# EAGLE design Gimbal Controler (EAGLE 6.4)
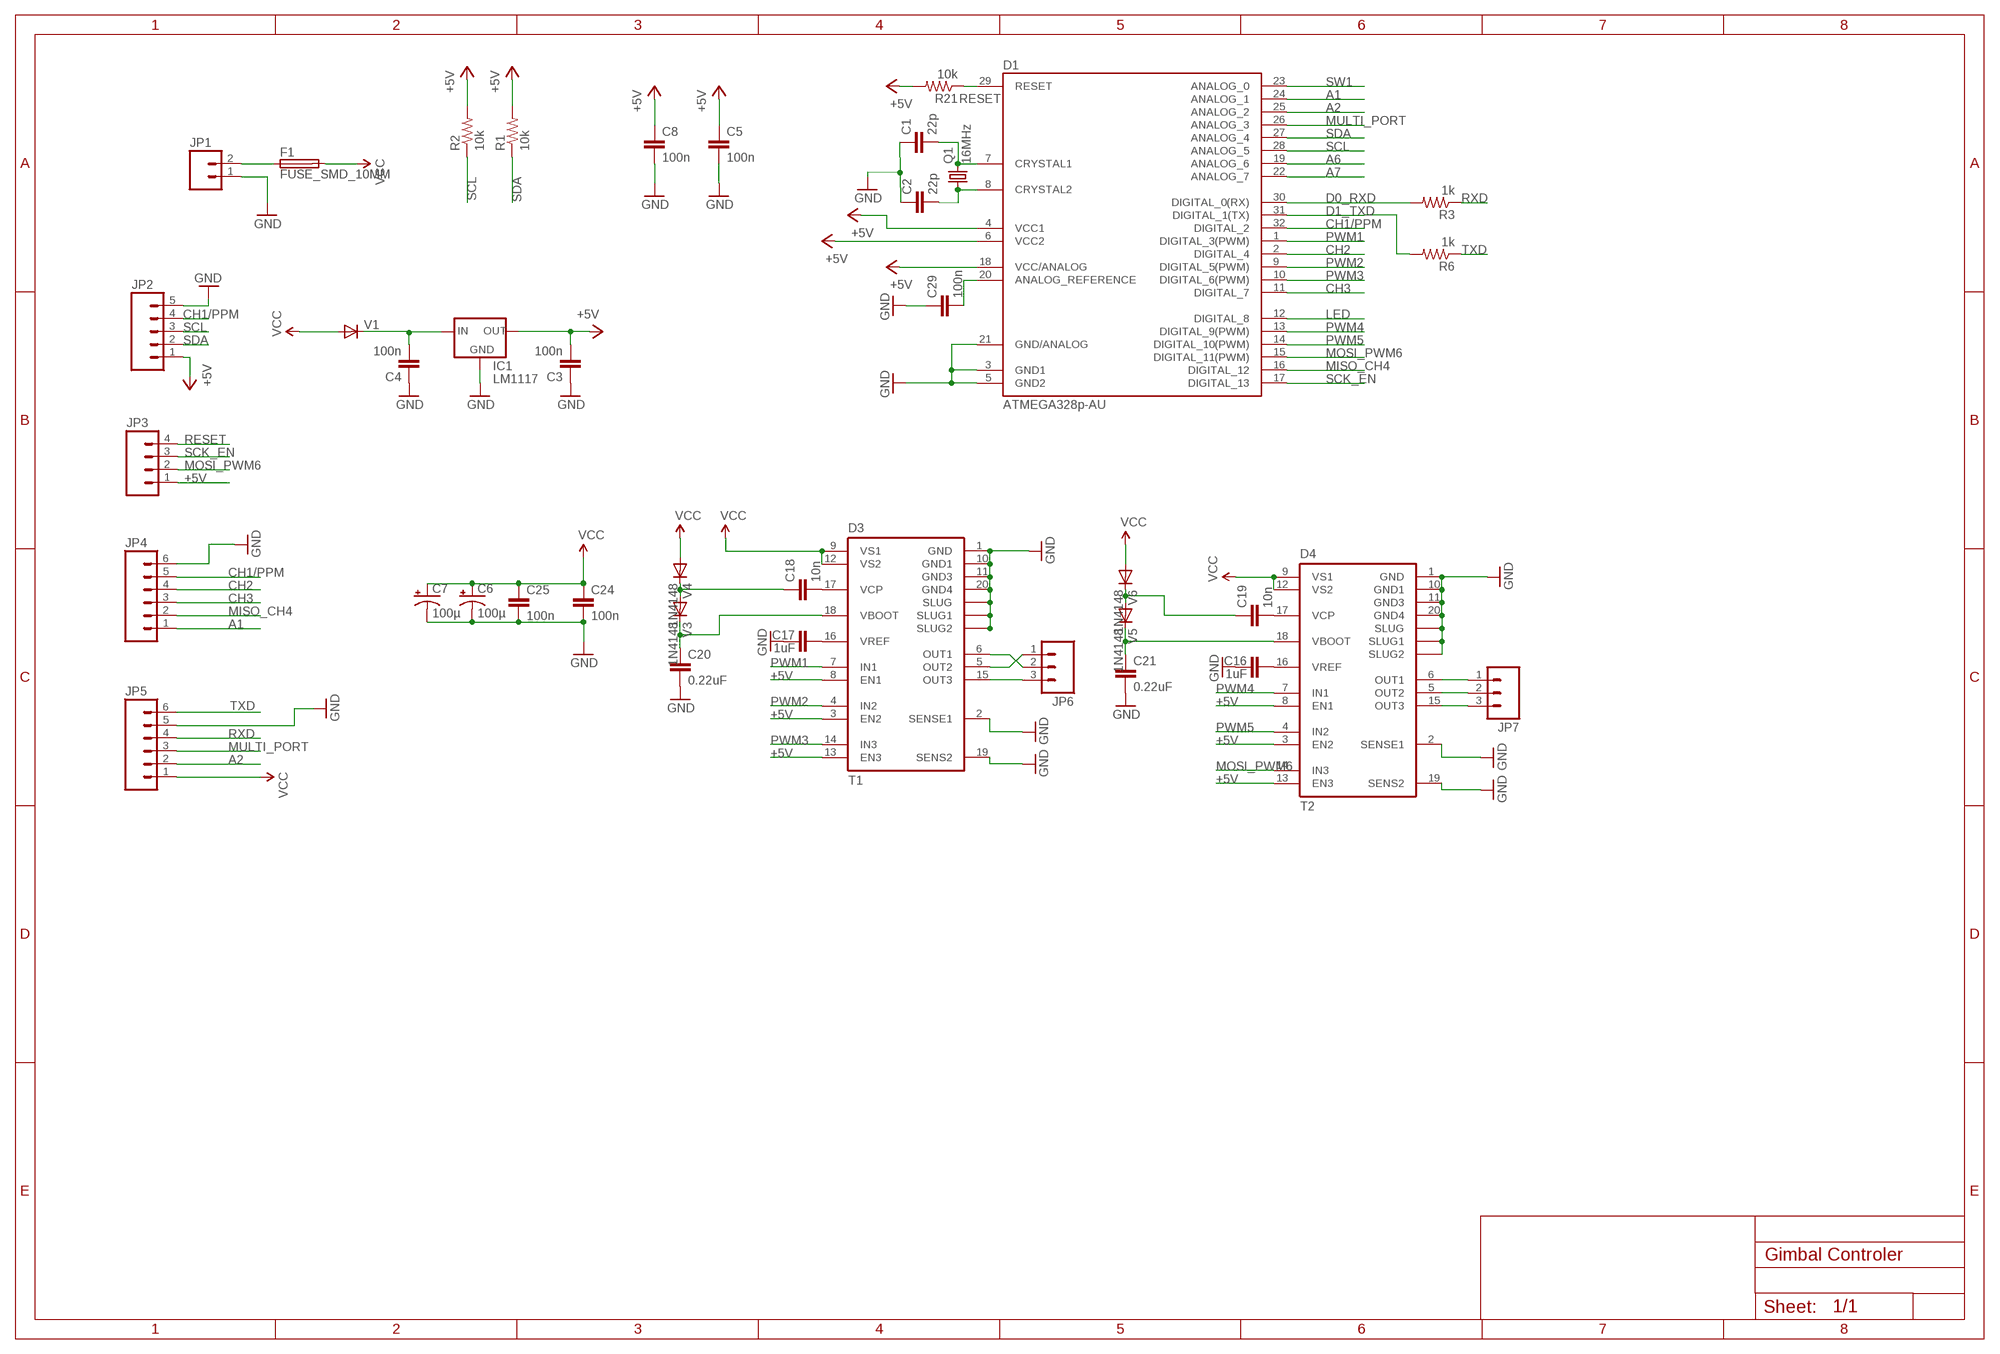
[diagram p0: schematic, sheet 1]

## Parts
C1  22p  CAP0805  [0805]
C2  22p  CAP0805  [0805]
C3  100n  CAP0805  [0805]
C4  100n  CAP0805  [0805]
C5  100n  CAP0805  [0805]
C6  100µ  CAP_POLD  [PANASONIC_D]
C7  100µ  CAP_POLD  [PANASONIC_D]
C8  100n  CAP0805  [0805]
C16  1uF  CAP0805  [0805]
C17  1uF  CAP0805  [0805]
C18  10n  CAP0805  [0805]
C19  10n  CAP0805  [0805]
C20  0.22uF  CAP0805  [0805]
C21  0.22uF  CAP0805  [0805]
C24  100n  CAP0805  [0805]
C25  100n  CAP0805  [0805]
C29  100n  CAP0805  [0805]
D1  ATMEGA328p-AU  ATMEGA168-AU  [TQFP32-08]
D3  T1  L6234  [SO20POWER2]
D4  T2  L6234  [SO20POWER2]
F1  FUSE_SMD_10MM  [SMD_FUSE_10MM]
IC1  LM1117  [SOT223]
JP1  M02PTH  [1X02]
JP2  M05PTH  [1X05]
JP3  M04PTH  [1X04]
JP4  M06SIP  [1X06]
JP5  M06SIP  [1X06]
JP6  M03PTH  [1X03]
JP7  M03PTH  [1X03]
Q1  16MHz  CRYSTALHC49S  [HC49/S]
R1  10k  RESISTOR0805-RES  [0805]
R2  10k  RESISTOR0805-RES  [0805]
R3  1k  RESISTOR0805-RES  [0805]
R6  1k  RESISTOR0805-RES  [0805]
R21  10k  RESISTOR0805-RES  [0805]
V1  DIODE-DO214AC  [DO214AC]
V3  1N4148  DIODE-MINIMELF  [MINIMELF]
V4  1N4148  DIODE-MINIMELF  [MINIMELF]
V5  1N4148  DIODE-MINIMELF  [MINIMELF]
V6  1N4148  DIODE-MINIMELF  [MINIMELF]

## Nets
+5V: C3.2 C5.1 C8.1 D1.4(VCC1) D1.6(VCC2) D1.18(VCC/ANALOG) D3.3(EN2) D3.8(EN1) D3.13(EN3) D4.3(EN2) D4.8(EN1) D4.13(EN3) IC1.2(OUT) JP2.1 JP3.1 R1.2 R2.2 R21.2
A1: D1.24(ANALOG_1) JP4.1
A2: D1.25(ANALOG_2) JP5.2
A6: D1.19(ANALOG_6)
A7: D1.22(ANALOG_7)
CH1/PPM: D1.32(DIGITAL_2) JP2.4 JP4.5
CH2: D1.2(DIGITAL_4) JP4.4
CH3: D1.11(DIGITAL_7) JP4.3
D0_RXD: D1.30(DIGITAL_0(RX)) R3.2
D1_TXD: D1.31(DIGITAL_1(TX)) R6.2
GND: C1.1 C2.1 C3.1 C4.1 C5.2 C6.- C7.- C8.2 C16.1 C17.1 C20.2 C21.2 C24.2 C25.2 C29.1 D1.3(GND1) D1.5(GND2) D1.21(GND/ANALOG) D3.1(GND) D3.2(SENSE1) D3.10(GND1) D3.11(GND3) D3.19(SENS2) D3.20(GND4) D3.SLUG1(SLUG2) D3.SLUG2(SLUG) D3.SLUG(SLUG1) D4.1(GND) D4.2(SENSE1) D4.10(GND1) D4.11(GND3) D4.19(SENS2) D4.20(GND4) D4.SLUG1(SLUG2) D4.SLUG2(SLUG) D4.SLUG(SLUG1) IC1.1(GND) JP1.1 JP2.5 JP4.6 JP5.5
LED: D1.12(DIGITAL_8)
MISO_CH4: D1.16(DIGITAL_12) JP4.2
MOSI_PWM6: D1.15(DIGITAL_11(PWM)) D4.14(IN3) JP3.2
MULTI_PORT: D1.26(ANALOG_3) JP5.3
N$3: F1.P$1 JP1.2
N$7: C16.2 D4.16(VREF)
N$8: C17.2 D3.16(VREF)
N$17: C18.2 D3.17(VCP)
N$18: C19.2 D4.17(VCP)
N$19: C19.1 V5.A V6.C
N$20: C21.1 D4.18(VBOOT) V5.C
N$21: D3.15(OUT3) JP6.3
N$23: D4.6(OUT1) JP7.1
N$24: D4.5(OUT2) JP7.2
N$25: D4.15(OUT3) JP7.3
N$27: D3.5(OUT2) JP6.1
N$28: D3.6(OUT1) JP6.2
N$38: C2.2 D1.8(CRYSTAL2) Q1.1
N$39: C1.2 D1.7(CRYSTAL1) Q1.2
N$40: C29.2 D1.20(ANALOG_REFERENCE)
PWM1: D1.1(DIGITAL_3(PWM)) D3.7(IN1)
PWM2: D1.9(DIGITAL_5(PWM)) D3.4(IN2)
PWM3: D1.10(DIGITAL_6(PWM)) D3.14(IN3)
PWM4: D1.13(DIGITAL_9(PWM)) D4.7(IN1)
PWM5: D1.14(DIGITAL_10(PWM)) D4.4(IN2)
RESET: D1.29(RESET) JP3.4 R21.1
RXD: JP5.4 R3.1
SCK_EN: D1.17(DIGITAL_13) JP3.3
SCL: D1.28(ANALOG_5) JP2.3 R2.1
SDA: D1.27(ANALOG_4) JP2.2 R1.1
SW1: D1.23(ANALOG_0)
TXD: JP5.6 R6.1
VBOOT1: C20.1 D3.18(VBOOT) V3.C
VCC: C6.+ C7.+ C24.1 C25.1 D3.9(VS1) D3.12(VS2) D4.9(VS1) D4.12(VS2) F1.P$2 JP5.1 V1.A V4.A V6.A
VCC_VI: C4.2 IC1.3(IN) V1.C
VCP1: C18.1 V3.A V4.C

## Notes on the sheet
- FTDI

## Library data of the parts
C1-C5 C8 C16-C21 C24 C25 C29 = SparkFun:CAP: Capacitor
C6 C7 = SparkFun:CAP_POL: Capacitor Polarized
D1 = Arduino-AVR:ATMEGA168
D3 D4 = L6234:L6234
F1 = f-lf-omniblok-s:FUSE_SMD_10MM
IC1 = v-reg-2:LM1117
JP1 = SparkFun:M02: Header 2
JP2 = SparkFun:M05: Header 5 Standard 5-pin 0.1" header. Use with straight break away headers (SKU : PRT-00116), right angle break away headers (PRT-00553), swiss pins (PRT-00743), machine pins (PRT-00117), and female headers (PRT-00115). Molex polarized connector foot print use with SKU : PRT-08230 with associated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
JP3 = SparkFun:M04: Header 4 Standard 4-pin 0.1" header. Use with straight break away headers (SKU : PRT-00116), right angle break away headers (PRT-00553), swiss pins (PRT-00743), machine pins (PRT-00117), and female headers (PRT-00115). Molex polarized connector foot print use with SKU : PRT-08231 with associated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
JP4 JP5 = SparkFun:M06: Header 6 Standard 6-pin 0.1" header. Use with straight break away headers (SKU : PRT-00116), right angle break away headers (PRT-00553), swiss pins (PRT-00743), machine pins (PRT-00117), and female headers (PRT-00115). Molex polarized connector foot print use with SKU : PRT-08094 with associated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
JP6 JP7 = SparkFun:M03: Header 3 Standard 3-pin 0.1" header. Use with straight break away headers (SKU : PRT-00116), right angle break away headers (PRT-00553), swiss pins (PRT-00743), machine pins (PRT-00117), and female headers (PRT-00115). Molex polarized connector foot print use with SKU : PRT-08232 with associated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
Q1 = crystal:CRYSTAL: CRYSTAL; OC_FARNELL: 1667008; OC_NEWARK: unknown
R1-R3 R6 R21 = SparkFun:RESISTOR: Resistor
V1 V3-V6 = diode:DIODE-: DIODE

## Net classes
0 default: width 0.406 mm, clearance 0.152 mm

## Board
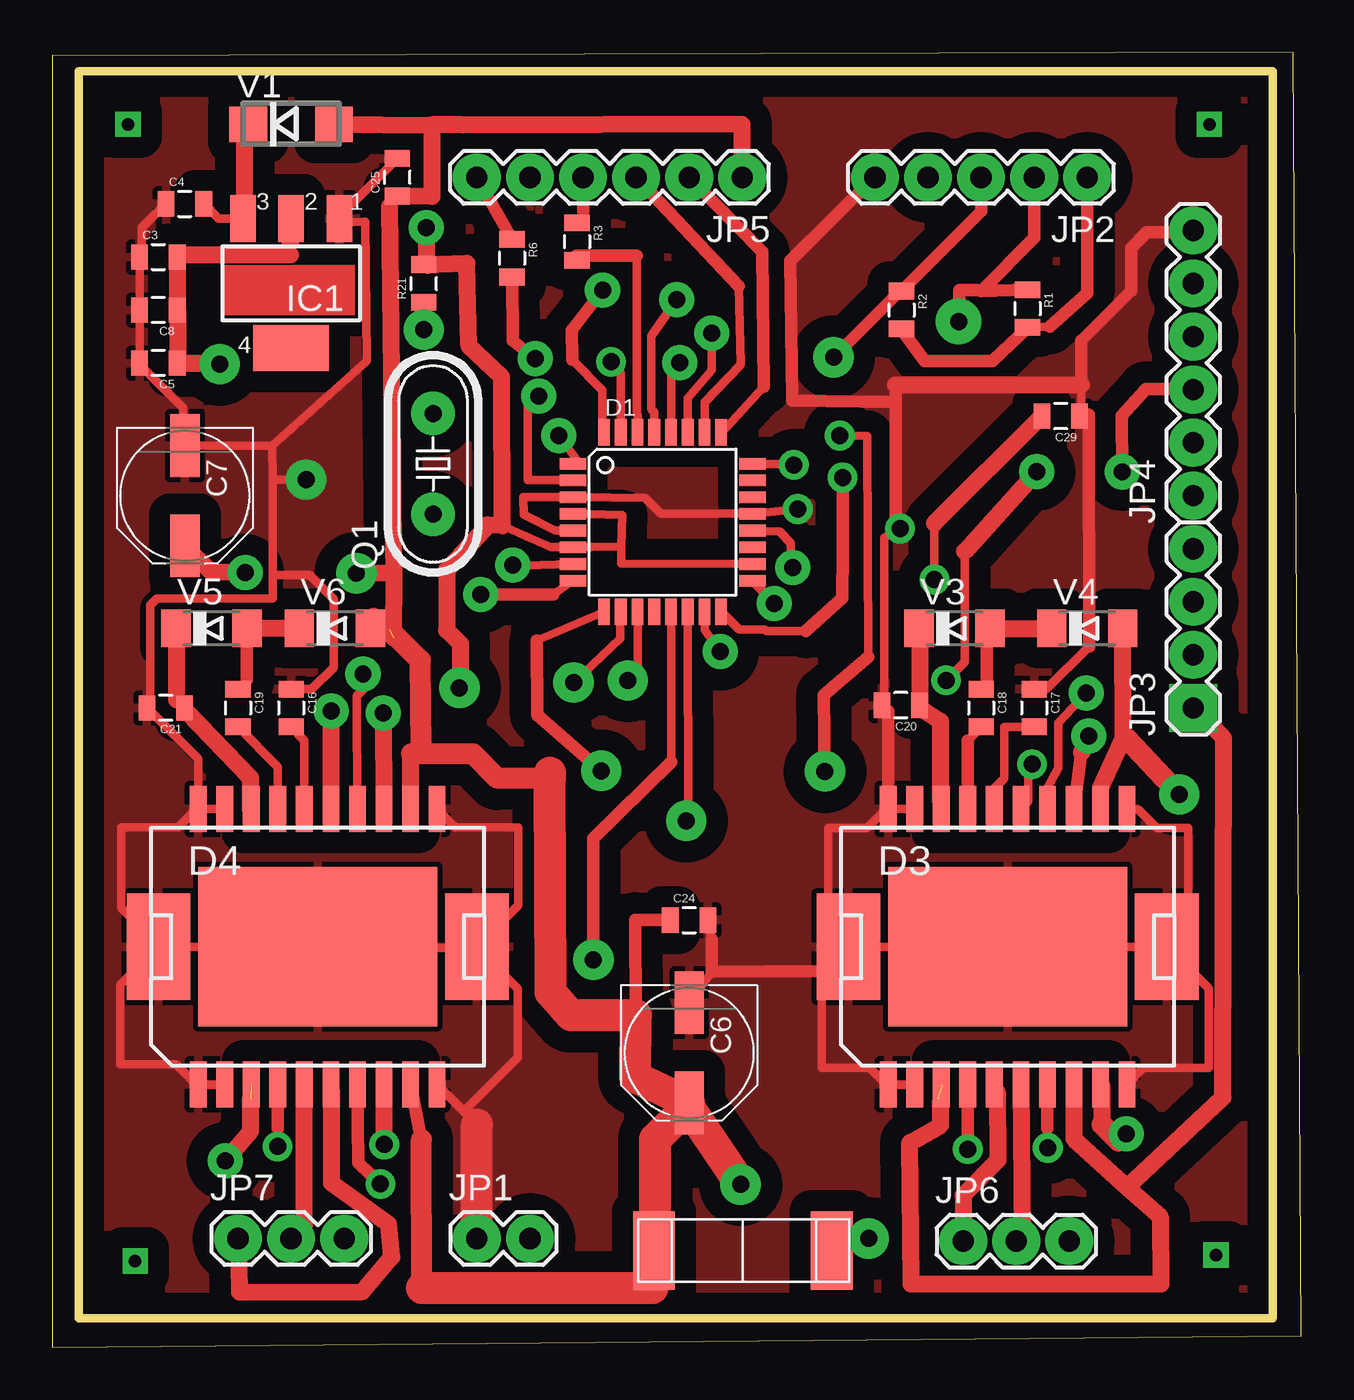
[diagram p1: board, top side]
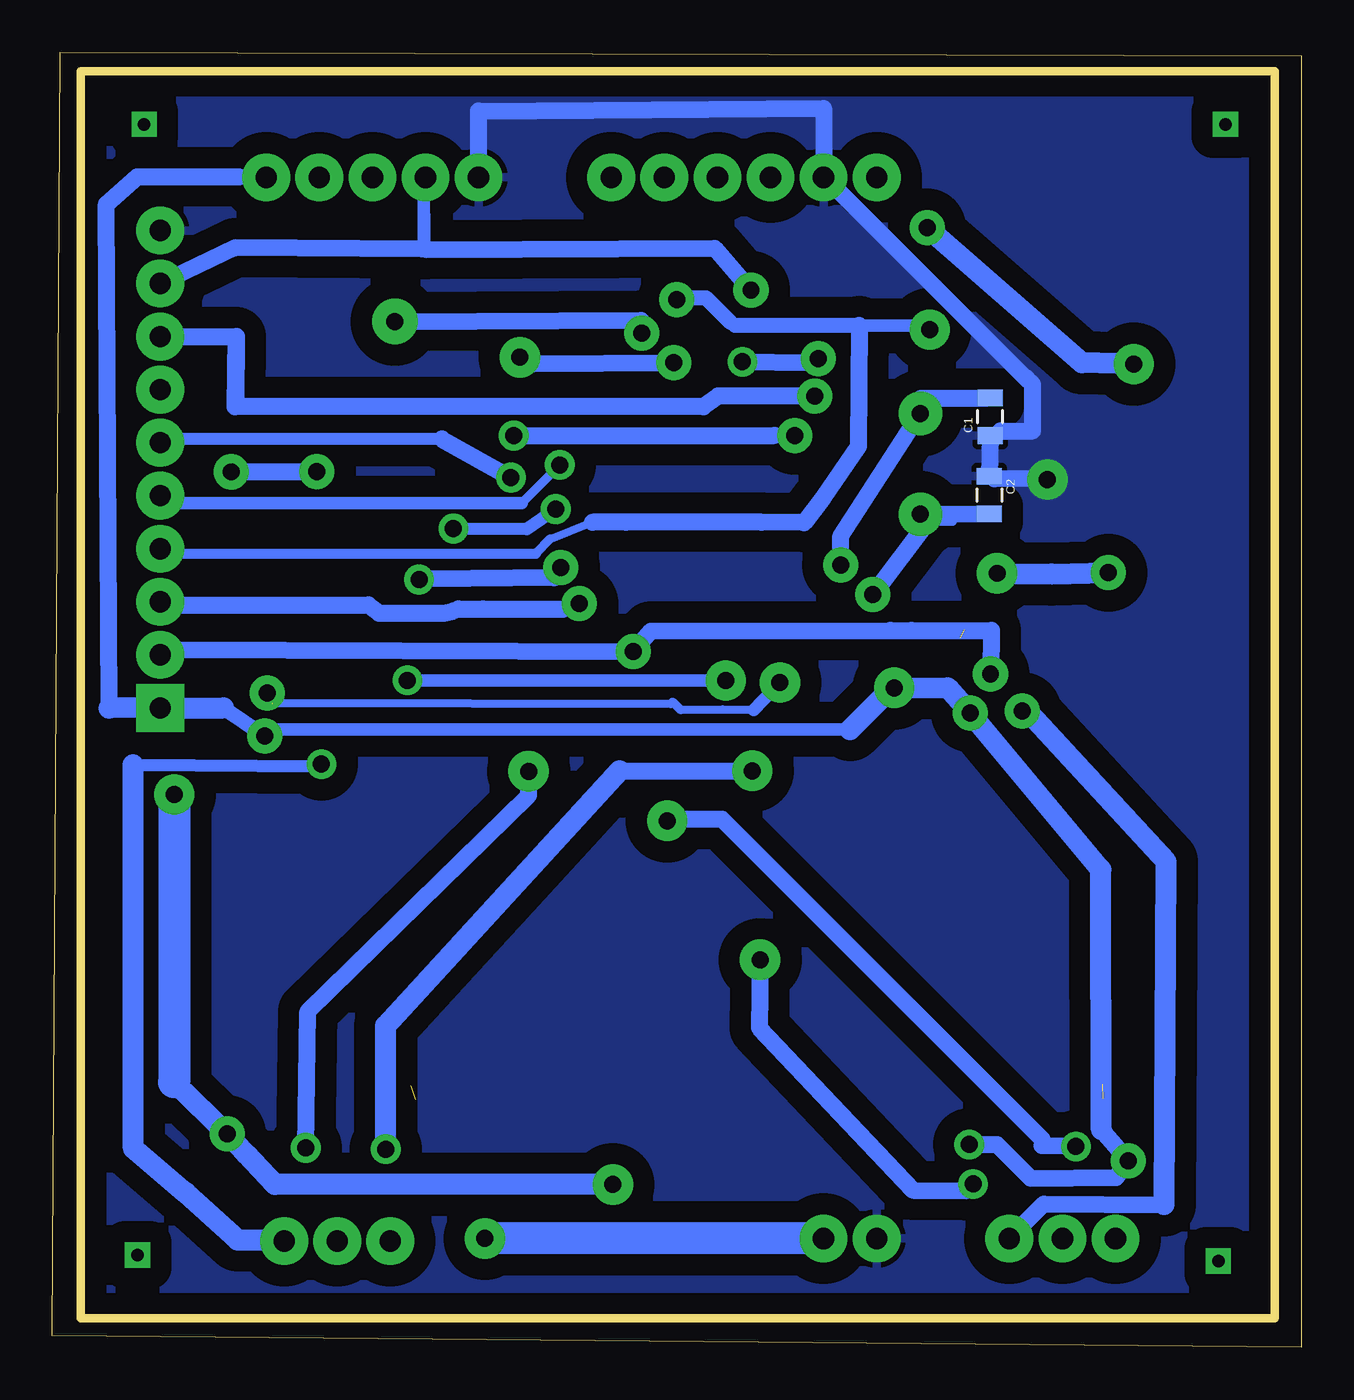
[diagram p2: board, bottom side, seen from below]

Size 59.77 x 62 mm. Coordinates in mm from the lower left corner, seen from the top.
Outline: 0,0 59.77,0.54 59.39,62 0,61.84 0,0
Outline: 58.42,61.09 58.42,1.4 1.27,1.4 1.27,61.09 58.42,61.09
Copper layers (1*16): Top 0.035mm / dielectric 1.5mm / Bottom 0.035mm
Design rules "default": minimum track width 10mil, minimum drill 32mil, track to track 12mil, track to pad 12mil, pad to pad 12mil, via to via 12mil, smd to smd 8mil, copper to edge 40mil, drill to drill 40mil, minimum pad ring 25mil, minimum via ring 12mil, stop-mask expansion 4mil, vias tented up to drill 0mil, thermal gap 10mil

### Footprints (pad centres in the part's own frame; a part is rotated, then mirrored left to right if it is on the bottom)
0805 = smd 0.8 x 1.2: 1 -0.9,0; 2 0.9,0
PANASONIC_D = smd 3 x 1.4: + 2.4,0; - -2.4,0
TQFP32-08 = smd 1.27 x 0.559: 1 -4.293,2.8; 2 -4.293,2; 3 -4.293,1.2; 4 -4.293,0.4; 5 -4.293,-0.4; 6 -4.293,-1.2; 7 -4.293,-2; 8 -4.293,-2.8; 17 4.293,-2.8; 18 4.293,-2; 19 4.293,-1.2; 20 4.293,-0.4; 21 4.293,0.4; 22 4.293,1.2; 23 4.293,2; 24 4.293,2.8 | smd 0.559 x 1.27: 9 -2.8,-4.293; 10 -2,-4.293; 11 -1.2,-4.293; 12 -0.4,-4.293; 13 0.4,-4.293; 14 1.2,-4.293; 15 2,-4.293; 16 2.8,-4.293; 25 2.8,4.293; 26 2,4.293; 27 1.2,4.293; 28 0.4,4.293; 29 -0.4,4.293; 30 -1.2,4.293; 31 -2,4.293; 32 -2.8,4.293
SO20POWER2 = smd 0.8 x 2.2: 1 -5.715,-6.6; 2 -4.445,-6.6; 3 -3.175,-6.6; 4 -1.905,-6.6; 5 -0.635,-6.6; 6 0.635,-6.6; 7 1.905,-6.6; 8 3.175,-6.6; 9 4.445,-6.6; 10 5.715,-6.6; 11 5.715,6.6; 12 4.445,6.6; 13 3.175,6.6; 14 1.905,6.6; 15 0.635,6.6; 16 -0.635,6.6; 17 -1.905,6.6; 18 -3.175,6.6; 19 -4.445,6.6; 20 -5.715,6.6 | smd 3.048 x 5.08: SLUG -7.62,0; SLUG2 7.62,0 | smd 11.43 x 7.62: SLUG1 0,0
SMD_FUSE_10MM = smd 2 x 3.75: P$1 4.25,0; P$2 -4.25,0
SOT223 = smd 1.219 x 2.235: 1 -2.311,-3.099; 2 0,-3.099; 3 2.311,-3.099 | smd 3.6 x 2.2: 4 0,3.099
1X02 = drill 1.016 pad 1.88: 1 0,0; 2 2.54,0
1X05 = drill 1.016 pad 1.88: 1 0,0; 2 2.54,0; 3 5.08,0; 4 7.62,0; 5 10.16,0
1X04 = drill 1.016 pad 1.88 square: 1 0,0 | drill 1.016 pad 1.88: 2 2.54,0; 3 5.08,0; 4 7.62,0
1X06 = drill 1.016 pad 1.88: 1 0,0; 2 2.54,0; 3 5.08,0; 4 7.62,0; 5 10.16,0; 6 12.7,0
1X03 = drill 1.016 pad 1.88: 1 0,0; 2 2.54,0; 3 5.08,0
HC49/S = drill 0.813: 1 -2.413,0; 2 2.413,0
DO214AC = smd 1.8 x 1.7: A 2.05,0; C -2.05,0
MINIMELF = smd 1.4 x 1.8: A 1.7,0; C -1.7,0

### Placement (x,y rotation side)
C1  14.89,44.55 90 bottom
C2  14.92,40.8 270 bottom
C3  5.08,52.2 0 top
C4  6.35,54.74 0 top
C5  5.08,47.12 180 top
C6  30.48,14.1 270 top
C7  6.35,40.77 270 top
C8  5.08,49.66 180 top
C16  11.43,30.61 270 top
C17  46.99,30.61 270 top
C18  44.45,30.61 270 top
C19  8.89,30.61 270 top
C20  40.61,30.73 180 top
C21  5.43,30.61 180 top
C24  30.48,20.45 0 top
C25  16.51,56.01 90 top
C29  48.26,44.58 180 top
D1  29.21,39.5 0 top
D3  45.72,19.18 0 top
D4  12.7,19.18 0 top
F1  33.05,4.64 0 top
IC1  11.43,50.93 180 top
JP1  20.32,5.21 0 top
JP2  49.53,56.01 180 top
JP3  54.61,30.61 90 top
JP4  54.61,40.77 90 top
JP5  33.02,56.01 180 top
JP6  43.59,5.08 0 top
JP7  8.89,5.21 0 top
Q1  18.22,42.29 90 top
R1  46.67,49.72 270 top
R2  40.64,49.66 270 top
R3  25.11,52.93 270 top
R6  22,52.13 270 top
R21  17.78,50.93 90 top
V1  11.43,58.55 0 top
V3  43.18,34.42 0 top
V4  49.53,34.42 0 top
V5  7.62,34.42 0 top
V6  13.53,34.42 0 top

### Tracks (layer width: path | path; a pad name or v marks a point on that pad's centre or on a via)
+5V  (via drill 0.81, 0.81 pad 1.68, 0.81 pad 1.93)  (2 unrouted)
  Top 0.406: 40.64,48.74 R2.2 | 47.73,48.86 R1.2 | 48.97,26.23 D3.13 | 42.6,12.52 D3.3 | 5.99,47.12 C5.1 | 5.99,49.66 C8.1 5.99,49.84 | 5.99,52.2 C3.2 6.17,52.3 | 11.41,52.9 IC1.2 11.49,53.81 | 11.41,52.3 11.38,52.84 | 21.54,39.33 22.71,38.8 23.85,38.3 D1.6 25.09,38.3 25.78,38.3 25.79,38.32 | R21.2 17.95,51.8 | 27.23,38.33 27.27,39.84 D1.4 | 25.79,38.32 27.23,38.33 | 27.23,38.33 27.23,38.34 25.79,38.32 | 27.23,38.33 27.23,37.52 D1.18 | 8.02,47.12 v8.02,47.07 | 41.04,9.8 41.14,9.84 | 42.51,11.75 42.39,11.88 | 19.53,31.61 v19.48,31.57
  Top 0.61: 40.64,48.74 41.75,47.22 44.99,47.22 R1.2 | 47.73,48.86 49.53,50.47 JP2.1 | 49.25,28.46 48.97,26.23
  Top 0.813: v49.6,29.25 49.25,28.46 | 41.04,9.8 41.1,3.02 53.05,3.02 53.02,6.27 51.45,7.65 | 51.45,7.65 48.9,9.98 D3.8 | JP3.1 56.06,29.16 56.03,11.94 51.45,7.65 | v15.89,9.71 15.87,10.49 D4.8 | v15.84,30.36 D4.13 | 5.99,49.66 5.99,47.12 8.02,47.12 | 5.99,49.84 5.99,52.2 | 11.38,52.84 11.41,52.9 | 6.17,52.3 11.41,52.3 | R21.2 19.84,51.89 19.93,47.94 21.51,46.46 21.54,39.33 20.84,39.36 18.88,37.21 18.88,34.33 19.53,33.69 19.53,31.61 | 17.95,51.8 v17.9,53.61 | 41.14,9.84 42.51,10.64 42.51,11.75 | v8.29,8.92 9.49,10.34 9.49,11.91
  Bottom 0.406: 50.83,56.04 JP2.1 | 54.62,30.63 JP3.1 | v15.89,9.71 15.87,9.19 | 49.4,29.57 49.84,29.13 v49.6,29.25 | 19.66,31.5 v19.48,31.57 | 8.87,8.13 v8.29,8.92
  Bottom 0.61: 21.59,29.57 49.4,29.57
  Bottom 0.711: 51.59,30.61 v49.6,29.25
  Bottom 0.813: 50.83,56.04 55.71,56.04 57.18,54.72 57.05,30.59 | 8.85,8.14 v8.29,8.92 9.56,10.41 | v15.89,9.71 14.57,9.71 12.95,8.1 8.87,8.13
  Bottom 1.016: JP3.1 51.59,30.61 | 54.62,30.63 57.05,30.59 | 9.56,10.41 9.6,22.87 v15.84,30.36 16.93,31.58 v19.48,31.57 | 19.66,31.5 21.59,29.57 | v8.02,47.07 10.5,47.13 v17.9,53.61
A1  (via drill 0.81)
  Top 0.406: v35.48,42.24 35.48,42.29 D1.24
  Bottom 0.406: 37.31,40.41 v35.48,42.24 | JP4.1 54.25,40.41
  Bottom 0.61: 54.25,40.41 37.31,40.41
A2
  Top 0.406: 34.06,45.98 32.03,43.79 D1.25
  Top 0.61: 34.06,45.98 33.97,52.46 JP5.2
CH1/PPM  (via drill 0.81 pad 1.68)
  Top 0.406: 24.89,47.28 26.31,45.82 26.31,43.87 26.39,43.79 D1.32
  Top 0.61: 24.89,47.28 24.86,48.7 v26.33,50.62
  Bottom 0.406: 41.88,52.55 JP2.4 42.09,55.91 42.08,52.58
  Bottom 0.813: v26.33,50.62 28.07,52.61 41.88,52.55 | JP4.5 51.02,52.64 42.08,52.58
CH2  (via drill 0.81 pad 1.68)
  Top 0.406: v23.28,45.54 22.76,45.14 22.76,41.5 D1.2
  Bottom 0.813: JP4.4 50.96,48.39 | 50.96,48.39 51,45.19 | v23.28,45.54 27.9,45.54 28.61,45.02 51.02,45.02 50.96,48.39
CH3  (via drill 0.81, 0.81 pad 1.68, 0.81 pad 1.93)
  Top 0.406: v27.54,31.92 28.02,32.28 D1.11 | v42.77,31.93 43.66,32.82 43.66,38.09 | 54.58,45.88 JP4.3
  Top 0.61: v51.21,41.91 51.18,44.61 52.32,45.88 54.58,45.88
  Top 0.813: v47.1,41.92 43.66,38.09
  Bottom 0.406: 28.12,31.93 v27.54,31.92
  Bottom 0.61: v42.77,31.93 28.12,31.93
  Bottom 0.813: v47.1,41.92 48.27,41.91 v51.21,41.91
D0_RXD
  Top 0.406: 25.07,52.25 25.05,52.04 R3.2 | 27.97,52.25 27.97,44.68 28.02,44.63 D1.30
  Top 0.61: 27.97,52.25 25.07,52.25
D1_TXD  (via drill 0.81, 0.81 pad 1.68)
  Top 0.406: v26.75,47.18 27.2,46.66 D1.31
  Top 0.61: v23.11,47.32 22.03,48.2 R6.2
  Bottom 0.813: v23.11,47.32 23.66,47.15 v26.75,47.18
GND  (via drill 0.81, 0.81 pad 1.93)
  Top 0.406: 49.62,33.54 47.57,31.52 46.99,31.52 C17.1 | 49.59,44.64 C29.1 49.25,44.76 49.25,46.08 | D3.SLUG2 55.35,17.17 55.35,13.39 52.22,13.39 51.44,12.6 D3.10 | D3.11 51.44,25.76 51.97,25.76 52.86,24.87 54.36,24.87 54.36,20.27 53.44,19.36 D3.SLUG2 | D3.SLUG2 D3.SLUG1 D3.SLUG | D1.5 24.08,39.09 22.57,39.87 22.54,40.7 24.05,40.69 D1.3 25.09,40.69 28.39,40.66 28.87,40.18 29.12,39.9 D1.21 33.68,39.9 v35.68,40.13 | 40.01,30.45 39.73,30.73 C20.2 39.83,30.91 39.83,38.76 v40.58,39.19 40.36,39.37 | D3.19 40.18,25.78 D3.20 39.83,25.68 39.01,24.87 37.14,24.87 37.14,18.64 D3.SLUG | 31.56,19.53 31.37,20.45 C24.2 | C6.- 31.56,17.98 | D3.2 D3.1 39.83,12.68 39.12,13.39 36.83,13.39 36.83,17.91 D3.SLUG | 36.65,18.01 D3.SLUG | 20.32,10.67 19.7,11.29 | 19.7,11.29 D4.10 | D4.SLUG2 22.3,21.16 22.3,24.89 19.28,24.89 18.41,25.76 D4.11 | 19.7,11.29 22.28,13.87 22.28,17.14 20.42,19 D4.SLUG2 | D4.20 6.98,28.17 4.55,30.61 C21.2 4.65,30.79 4.7,30.84 4.7,35.54 5,35.84 10.54,35.84 10.54,37.02 | D4.19 7.16,25.78 D4.20 | D4.2 D4.1 6.81,12.68 5.94,13.54 3.25,13.54 3.25,17.35 D4.SLUG | D4.20 6.81,25.68 6.02,24.89 3.3,24.89 3.3,21.03 4.98,19.36 D4.SLUG | D4.SLUG D4.SLUG1 12.88,19.13 20.12,19.13 D4.SLUG2 | C4.1 5.44,54.74 4.29,53.59 4.29,52.38 C3.1 4.19,52.2 4.19,49.84 C8.2 4.19,49.66 4.19,47.12 C5.2 4.29,46.94 6.27,44.96 6.27,43.36 C7.- 6.35,43.16 10.53,43.17 | C25.2 16.51,56.9 13.74,54.13 IC1.1 13.84,53.85 14.99,53.88 15.05,47.21 10.53,43.17 | 10.54,41.54 10.54,37.02 | 10.53,43.17 10.54,41.54 | 11.43,31.52 C16.1 12.42,31.51 13.46,32.54 13.46,35.81 12.32,36.96 10.6,36.96 10.54,37.02 | v12.15,41.54 10.54,41.54
  Top 0.406: 40.31,45.26 40.36,46.08 | 54.52,53.37 JP4.6
  Top 0.61: 49.59,44.64 49.62,33.54 | 49.25,46.08 49.25,48.2 51.63,50.58 51.63,52.61 52.39,53.37 54.52,53.37 | D3.20 40.01,30.45 | 31.56,19.53 31.56,17.98 36.65,18.01 | 40.36,39.37 40.36,46.08 | 40.31,45.26 35.41,45.32 35.31,52.01 JP2.5
  Top 0.813: 40.36,46.08 49.25,46.08
  Top 1.524: JP1.1 20.32,10.67
  Bottom 0.406: v12.15,41.54 11.88,41.57 | 14.68,41.58 C2.1 | 13.16,46.41 13.18,46.41 | 22.68,55.91 JP5.5 | 14.4,43.87 C1.1
  Bottom 0.61: v35.68,40.13 37.06,39.16 v40.58,39.19
  Bottom 0.813: JP5.5 22.86,59.31 39.37,59.18 JP2.5 | C1.1 C2.1 | 11.88,41.57 14.68,41.58 | 13.18,46.41 22.68,55.91 | 13.16,46.41 12.85,46.1 12.85,43.87 14.4,43.87
  pour Bottom (isolate 1.016): 1.43,61.02 58.23,61.12 58.42,60.93 58.45,1.37 1.33,1.27 1.24,1.37 1.24,60.83
  pour Top (isolate 1.016): 58.36,61.15 58.42,58.71 58.32,4.03 58.36,1.62 1.4,1.59 1.21,1.4 1.3,61.09
  pour Bottom (isolate 1.016): 58.39,61.02 58.36,57.88 58.36,57.4 58.42,41.91 58.45,1.49 58.36,1.46 1.4,1.52 0.86,60.99 2,60.99
MISO_CH4  (via drill 0.81)
  Top 0.406: 36.07,34.29 34.16,34.29 34.09,34.37 32.87,34.37 32.03,35.2 D1.16
  Top 0.61: 36.07,34.29 37.81,35.87 37.82,38.12 v37.82,41.63
  Bottom 0.406: JP4.2 54.05,43.51
  Bottom 0.61: 54.05,43.51 41.13,43.48
  Bottom 0.813: 41.13,43.48 v37.82,41.63
MOSI_PWM6  (via drill 0.81 pad 1.68)
  Top 0.406: v31.97,33.31 31.22,34.34 D1.15 | D4.14 14.57,31.18 14.87,31.49 v14.87,32.23
  Bottom 0.406: 18.64,34.32 19.67,34.32 | JP3.2 54.1,33.4
  Bottom 0.813: 18.64,34.32 31.12,34.28 v31.97,33.31 54.1,33.4 | 19.67,34.32 14.83,34.32 v14.87,32.23
MULTI_PORT
  Top 0.406: 32.84,50.79 32.94,47.05 31.22,45.24 D1.26
  Top 0.61: JP5.3 32.84,50.79
N$1  (via drill 0.6)
  other vias: 3.97,4.13
N$2  (via drill 0.6)
  other vias: 55.69,4.41
N$3  (via drill 0.81 pad 1.93)
  Top 0.406: v39.07,5.21 F1.P$1
  Bottom 1.524: JP1.2 v39.07,5.21
N$4  (via drill 0.6)
  other vias: 55.37,58.55
N$5  (via drill 0.6)
  other vias: 3.62,58.55
N$7
  Top 0.406: D4.16 12.06,29.06 11.43,29.69 C16.2
N$8
  Top 0.406: D3.16 45.09,26.75 45.57,27.23 45.57,29.69 46.99,29.69 C17.2
N$17
  Top 0.406: 43.82,29.06 44.45,29.69 C18.2
  Top 0.61: D3.17 43.82,29.06
N$18
  Top 0.406: D4.17 10.79,27.79 8.89,29.69 C19.2
N$19
  Top 0.406: 9.32,31.94 C19.1
  Top 0.61: V5.A 9.32,31.94
  Top 0.813: V6.C V5.A
N$20
  Top 0.406: 5.94,30.99 C21.1 6.43,30.43 | 5.94,34.42 V5.C | 9.49,25.72 D4.18
  Top 0.813: 5.94,34.42 5.94,30.99 | 9.49,25.72 9.49,27.27 6.43,30.43
N$21  (via drill 0.81)
  Top 0.406: v46.89,27.91 46.71,27.74 46.71,26.14 D3.15
  Bottom 0.406: 46.99,27.81 v46.89,27.91 | 53.41,7.4 53.37,7.4 | 48.74,5.14 JP6.3
  Bottom 0.61: 55.91,27.88 46.99,27.81
  Bottom 1.016: 55.91,27.88 55.89,9.51 53.41,7.4 | 53.37,7.4 50.9,5.14 48.74,5.14
N$23
  Top 0.406: 13.37,12.25 D4.6
  Top 0.813: 13.37,12.25 13.37,7.85 16.1,5.89 16.26,4.33 14.85,2.67 8.95,2.63 JP7.1
N$24
  Top 0.813: D4.5 12.06,5.84 JP7.2
N$25  (via drill 0.81 pad 1.68)
  Top 0.406: 13.33,26.17 D4.15 | 13.33,27.9 13.33,27.84
  Top 0.813: 13.33,27.84 13.33,26.17 | 13.33,27.9 13.33,29.24 v13.34,30.45
  Bottom 0.406: 13.02,30.35 v13.34,30.45
  Bottom 0.813: 6.56,6.83 12.32,6.86 JP7.3
  Bottom 1.016: 13.02,30.35 6.46,23.25 6.56,6.83
N$27
  Top 0.406: 45.22,12.25 D3.5
  Top 0.813: 45.22,12.25 45.25,8.96 43.59,7.27 JP6.1
N$28
  Top 0.406: 46.42,5.3 JP6.2
  Top 0.813: D3.6 46.42,5.3
N$38  (via drill 0.81 pad 1.68)
  Top 0.406: 23.97,36.04 D1.8
  Top 0.61: v20.51,36.04 23.97,36.04
  Bottom 0.406: 15.22,39.91 15.08,39.92 C2.2 | 17.88,39.52 16.69,39.52 Q1.1
  Bottom 0.813: Q1.1 15.22,39.91 | 17.88,39.52 v20.51,36.04
N$39  (via drill 0.81 pad 1.68)
  Top 0.406: v22.03,37.45 22.57,37.43 D1.7
  Bottom 0.406: Q1.2 18.19,45.43 | 15.08,45.43 C1.2
  Bottom 0.813: 18.19,45.43 15.08,45.43 | v22.03,37.45 22.06,38.78 Q1.2
N$40  (via drill 0.81, 0.81 pad 1.68)
  Top 0.406: v42.22,36.75 42.22,39.45 | v35.43,37.34 35.34,38.02 35.34,38.49 34.81,39.06 D1.20 | 47.35,44.58 C29.2
  Top 0.813: 42.22,39.45 47.35,44.58
  Bottom 0.406: 41.74,36.79 v42.22,36.75
  Bottom 0.813: 41.74,36.79 35.76,36.85 v35.43,37.34
PWM1  (via drill 0.81, 0.81 pad 1.68, 0.81 pad 1.93)
  Top 0.406: v24.24,43.64 25.09,42.49 24.92,42.32 D1.1 | v37.69,43.65 39.01,43.63 39.04,33.04 | 47.62,10.49 v47.64,9.55
  Top 0.61: 39.04,33.04 36.91,31.23 v36.98,27.57 | D3.7 47.62,10.49
  Bottom 0.406: 25.22,43.65 v24.24,43.64
  Bottom 0.813: v37.69,43.65 25.22,43.65 | v36.98,27.57 36.98,26.42 47.54,16.08 v47.64,9.55
PWM2  (via drill 0.81, 0.81 pad 1.93)
  Top 0.406: 23.19,33.85 26.39,35.2 D1.9
  Top 0.61: 23.19,33.85 23.22,30.27 v26.28,27.6 | D3.4 v43.82,9.49
  Bottom 0.813: 32.63,27.6 v26.28,27.6
  Bottom 1.016: 32.63,27.6 43.82,15.39 v43.82,9.49
PWM3  (via drill 0.81 pad 1.68, 0.81 pad 1.93)  (1 unrouted)
  Top 0.406: v24.95,31.83 27.17,33.92 D1.10 | v49.49,31.32 48.14,29.88 48.14,27.74 47.62,26.75 D3.14
  Bottom 0.406: v49.49,31.32 49.24,30.83 | 26.2,30.51 27.69,30.54 29.69,30.51 30.07,30.89 30.1,30.89 30.19,30.81 49.27,30.84
  Bottom 0.61: 26.2,30.51 v24.95,31.83
PWM4  (via drill 0.81, 0.81 pad 1.93)
  Top 0.406: 29.62,28.02 D1.13
  Top 0.61: 29.62,28.02 25.9,24.36 v25.9,18.55 | v15.7,7.82 14.64,8.82 D4.7
  Bottom 0.813: v25.9,18.55 25.93,15.29 18.57,7.52 16.03,7.49 v15.7,7.82
PWM5  (via drill 0.81, 0.81 pad 1.93)
  Top 0.406: v30.34,25.2 30.38,25.2 arc90 30.45,25.27 D1.14 | 10.79,10.49 v10.78,9.61
  Top 0.61: D4.4 10.79,10.49
  Bottom 0.406: 12.4,9.65 12.4,9.96 | 30.27,25.27 v30.34,25.2
  Bottom 0.813: v10.78,9.61 12.4,9.65 | 12.4,9.96 27.72,25.27 30.27,25.27
RESET  (via drill 0.81 pad 1.68, 0.81 pad 1.93)
  Top 0.406: v29.88,50.16 28.68,48.41 28.68,44.91 28.8,44.78 D1.29
  Top 0.813: v17.78,48.72 R21.1
  Bottom 0.406: 18.62,48.92 v17.78,48.72 | 54.36,37.97 JP3.4 | 36.65,38.01 35.94,38.72 36.03,38.65 33.91,39.5 | 27.11,48.92 27.24,49.05 27.3,49.05 | 29.81,50.23 v29.88,50.16
  Bottom 0.508: 36.65,38.01 54.36,37.97
  Bottom 0.61: 21.16,48.92 18.62,48.92
  Bottom 0.711: 21.16,48.92 27.11,48.92 | 27.3,49.05 28.48,50.23 29.81,50.23
  Bottom 0.813: 33.91,39.5 32.32,39.5 25.82,39.5 23.79,39.47 22.87,40.68 21.19,43.12 21.16,48.92
RXD
  Top 0.406: 25.4,54.38 25.21,53.78 R3.1
  Top 0.61: JP5.4 25.4,54.38
SCK_EN  (via drill 0.81 pad 1.68)
  Top 0.406: v34.54,35.6 33.5,36.68 D1.17
  Bottom 0.406: 39.15,35.34 39.11,35.34 | 40.56,35.25 40.34,35.34 | JP3.3 54.46,35.54
  Bottom 0.813: v34.54,35.6 35.33,35.34 39.11,35.34 | 40.34,35.34 39.15,35.34 | 54.46,35.54 44.65,35.54 44.13,35.15 41.02,35.15 40.56,35.25
SCL  (via drill 0.81 pad 1.68, 0.81 pad 1.93)
  Top 0.406: 40.64,50.57 R2.1 40.46,50.47 | v30.02,47.14 29.62,46.76 D1.28
  Top 0.61: 40.64,50.57 44.45,54.38 JP2.3 | 40.46,50.47 v37.39,47.4
  Bottom 0.813: v30.02,47.14 36.76,47.08 v37.39,47.4
SDA  (via drill 0.81 pad 1.68, 0.81 pad 2.18)
  Top 0.406: v31.56,48.55 31.56,46.79 30.4,45.44 D1.27 | 44.27,50.6 R1.1
  Top 0.61: JP2.2 46.99,53.11 44.45,50.57 R1.1 | v43.38,49.11 43.41,50.6 44.27,50.6
  Bottom 0.813: v31.56,48.55 31.6,49.17 v43.38,49.11
TXD
  Top 0.61: JP5.6 R6.1
VBOOT1
  Top 0.406: C20.1 41.61,30.56 | 41.5,34.42 V3.C | 42.51,26.14 D3.18
  Top 0.813: 41.5,34.42 C20.1 | 42.51,26.14 42.51,29.97 41.61,30.56
VCC  (via drill 0.81 pad 1.68, 0.81 pad 1.93)  (1 unrouted)
  Top 0.406: C25.1 16.43,54.91 16.14,54.62 | 19.63,58.52 19.61,58.52 | 18.16,58.52 18.17,57.44 | 17.65,28.69 17.15,28.45 17.18,28.42 | 16.13,34.37 V6.A | 51.26,29.18 51.26,29.03 51.41,29.15 | D3.12 50.16,26.75 | V4.A | 29.57,20.45 C24.1 | 30.48,11.71 C6.+ | 28.72,2.83 28.75,5.21 F1.P$2 28.85,5.38 | D4.9 | 30.4,11.51 C6.+ | 30.56,11.35 C6.+ | D3.9 50.23,12.51 | 51.03,9.87 v51.4,10.22 | 21.3,27.24 21.37,27.24
  Top 0.61: 29.57,20.45 27.9,20.46 27.93,15.9 | 17.66,9.93 D4.9
  Top 0.813: C25.1 18.17,55.09 18.17,57.44 18.17,58.52 V1.A | 19.61,58.52 18.16,58.52 | 19.63,58.52 33.02,58.55 JP5.1 | D4.12 17.15,28.45 | v9.23,37.08 7.62,37.12 C7.+ | 51.26,29.03 V4.A | 50.16,26.75 51.26,29.18 | 16.36,37.08 16.33,33.96 15.37,34.99 | 16.36,37.08 16.33,38.45 16.14,54.62 | 50.23,12.51 50.23,10.67 | v14.55,37.05 16.36,37.08
  Top 1.016: 16.13,34.37 17.62,32.88 17.65,28.69 | 51.41,29.15 v53.94,26.47 | 17.69,2.83 17.66,9.93 | 50.23,10.67 51.03,9.87 | 17.18,28.42 20.13,28.42 21.3,27.24 | 21.37,27.24 23.82,27.24
  Top 1.524: 30.48,11.71 27.9,12.93 27.93,15.9 24.82,15.9 23.85,16.99 23.82,27.24 23.82,27.5 | 17.69,2.83 19.6,2.83 28.72,2.83 | 30.4,11.51 28.85,9.96 28.85,5.38 | 30.56,11.35 v32.94,7.79
  Bottom 1.016: v9.23,37.08 11.95,37.03 v14.55,37.05 | 53.94,12.69 v51.4,10.22 50.5,9.26 49.12,7.79 v32.94,7.79
  Bottom 1.524: v53.94,26.47 53.94,12.69
VCC_VI
  Top 0.406: C4.2 7.26,54.74 7.98,54.03 IC1.3 9.22,54.2 | 9.22,58.4 V1.C
  Top 0.813: 9.22,54.2 9.22,58.4
VCP1
  Top 0.406: 44.73,31.93 44.45,31.52 C18.1 | 44.73,34.42 V3.A
  Top 0.61: 44.73,34.42 44.73,31.93
  Top 0.813: V3.A V4.C
(copper drawn outside any net)
  shapes: Top area x1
